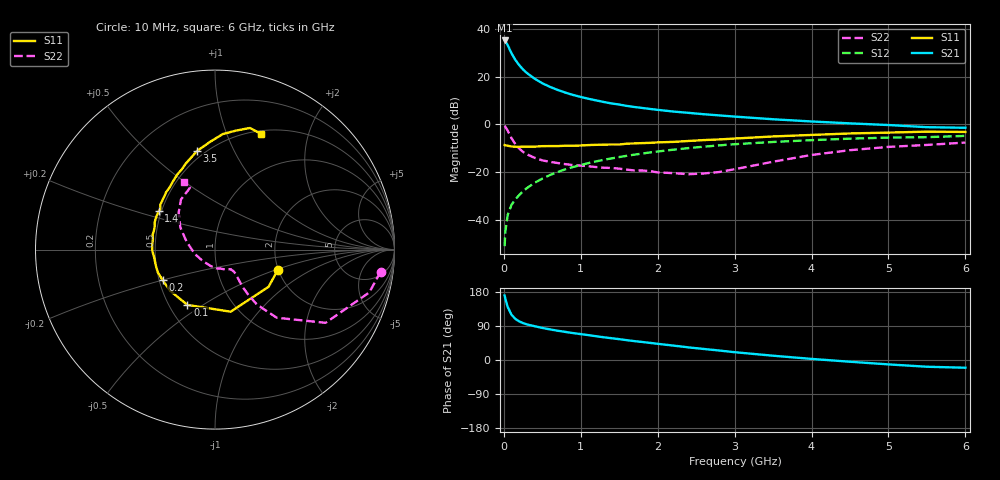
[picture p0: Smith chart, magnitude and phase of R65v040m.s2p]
! Infineon Technologies  Discrete & RF Semiconductors
! BFR193
! Si NPN RF Bipolar Junction Transistor in SOT23
! VCE = 5 V  IC = 40 mA
! Common Emitter S-Parameters:  April  1999
# GHz  S  MA  R  50
!  f  S11  S21  S12  S22
! GHz  MAG  ANG  MAG  ANG  MAG  ANG  MAG  ANG
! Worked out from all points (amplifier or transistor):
!   36 points, 10 MHz to 6 GHz, reference 50 ohm
!   highest |S21| = 35.2 dB at 10 MHz (marker M1)
!   |S21| within 3 dB of that: start of sweep to 64.8 MHz
!   unconditionally stable (mu >= 1): 440.8 MHz to 1.973 GHz
!   at 250 MHz: K = 0.92, MSG = 25.5 dB, |S12| = -28.0 dB
!   at 1.4 GHz: K = 1.02, MAG = 10.6 dB, |S12| = -14.3 dB
!   at 6 GHz: K = 0.95, MSG = 1.7 dB, |S12| = -4.8 dB
!   lowest NFmin = 1.85 dB at 50 MHz
!   S11 on the Smith chart (normalised r, x): 10 MHz: 1.99, -0.52; 100 MHz: 0.62, -0.43; 200 MHz: 0.52, -0.20; 1.4 GHz: 0.48, +0.24; 3.5 GHz: 0.45, +0.73; 6 GHz: 0.53, +1.33
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0.01  0.3678 -17.8  57.46 170.3  0.0028 82.9  0.9311 -7.6
0.02  0.3634 -34.7  55.69 161.1  0.0057 78.4  0.8922 -15.5
0.05  0.3569 -75.8  45.66 139.9  0.0126 71.1  0.739 -33.5
0.1  0.3444 -116.5  30.92 119.4  0.0206 66.7  0.5125 -47.8
0.15  0.3395 -137.6  22.42 108.3  0.0269 67.8  0.3842 -52.7
0.2  0.3378 -149.9  17.44 101.9  0.033 69.7  0.3117 -53.6
0.25  0.343 -158.2  14.14 97.4  0.0398 71.1  0.2651 -53.5
0.3  0.3416 -164.1  11.92 94.0  0.0462 72.5  0.2359 -52.7
0.4  0.3416 -172.4  9.08 89.1  0.0597 73.1  0.1993 -51.1
0.5  0.3498 -179.2  7.285 84.6  0.0729 73.3  0.1762 -49.7
0.6  0.3509 175.8  6.112 80.8  0.0867 72.8  0.1638 -49.4
0.7  0.3508 170.4  5.278 77.2  0.1006 72.0  0.1549 -49.8
0.8  0.3573 166.5  4.633 74.1  0.1143 71.0  0.1465 -50.8
0.9  0.3564 162.4  4.138 71.1  0.1277 70.0  0.1404 -51.2
1.1  0.3685 156.1  3.443 65.5  0.1546 67.6  0.1325 -55.8
1.4  0.3796 145.8  2.75 57.5  0.1938 63.6  0.1221 -63.5
1.7  0.3994 137.7  2.315 49.8  0.2326 59.4  0.1082 -75.0
2.2  0.4295 126.0  1.862 38.1  0.2946 52.0  0.0952 -103.6
3.5  0.5587 100.3  1.281 11.3  0.4282 31.8  0.165 164.1
4.5  0.6456 86.1  1.051 -4.6  0.5024 17.7  0.288 134.7
5.5  0.705 74.0  0.874 -17.8  0.54 3.9  0.3711 112.1
6  0.6943 68.5  0.849 -20.4  0.5742 0.0  0.4162 114.4
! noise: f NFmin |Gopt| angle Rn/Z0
0.05  1.85  0.32  179  0.08
0.25  1.87  0.35  -178  0.08
0.45  1.95  0.38  -175  0.09
0.65  2.02  0.42  -171  0.1
0.9  2.13  0.48  -167  0.11
